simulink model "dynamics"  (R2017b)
settings: Solver=VariableStepAuto  StartTime=0.0  StopTime=10.0  RelTol=1e-3
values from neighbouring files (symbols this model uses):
  ModelInit_AngEuler = [0, 0, 0]    [Init_control.m]    (also in Init.m)
  ModelInit_PosE = [0, 0, -100]    [Init_control.m]    (also in Init.m = [0, 0, 0])
  ModelInit_Rads = 0    [Init.m]    (also in Init_control.m = 557.142)
  ModelInit_RateB = [0, 0, 0]    [Init_control.m]    (also in Init.m)
  ModelInit_VelB = [0, 0, 0]    [Init_control.m]    (also in Init.m)
  ModelParam_envGravityAcc = 9.8    [Init.m]
  ModelParam_motorCr = 1148    [Init.m]    (also in Init_control.m)
  ModelParam_motorJm = 0.0001287    [Init.m]    (also in Init_control.m)
  ModelParam_motorT = 0.02    [Init.m]    (also in Init_control.m)
  ModelParam_motorWb = -141.4    [Init.m]    (also in Init_control.m)
  ModelParam_rotorCm = 1.779e-07    [Init.m]    (also in Init_control.m)
  ModelParam_rotorCt = 1.105e-05    [Init.m]    (also in Init_control.m)
  ModelParam_uavCCm = [0.01 0.01 0.0055]    [Init.m]
  ModelParam_uavCd = 0.073    [Init.m]
  ModelParam_uavJ = [ModelParam_uavJxx, 0, 0;     0, ModelParam_uavJyy, 0;     0, 0, ModelParam_uavJzz]    [Init.m]    (also in Init_control.m)
  ModelParam_uavMass = 1.4    [Init.m]    (also in Init_control.m)
  ModelParam_uavR = 0.225    [Init.m]    (also in Init_control.m)
undefined symbols (not defined in the file or in its folder): Column, D, vector
libraries: sharedutil x2

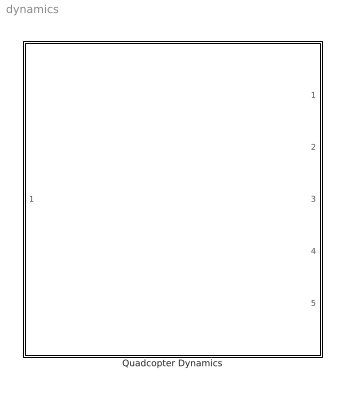
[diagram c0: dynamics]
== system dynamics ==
  Quadcopter Dynamics : Subsystem

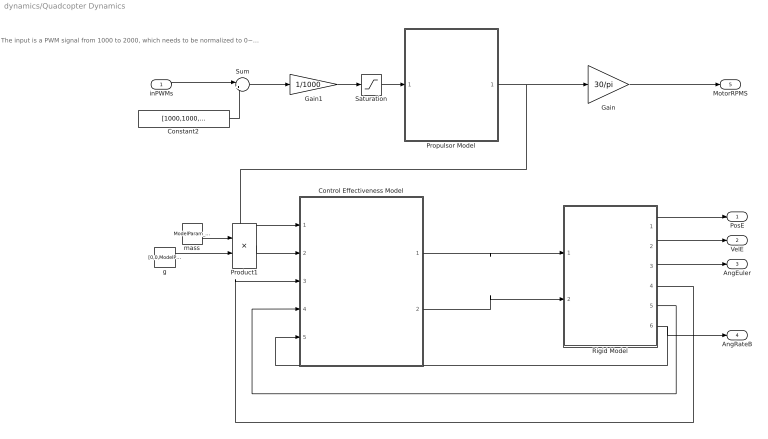
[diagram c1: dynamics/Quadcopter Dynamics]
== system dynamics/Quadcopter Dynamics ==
  note: The input is a PWM signal from 1000 to 2000, which needs to be normalized to 0~1.
  inPWMs : Inport
  Constant2 : Constant  Value=[1000,1000,1000,1000]
  Control Effectiveness Model : Subsystem
  Gain : Gain  Gain=30/pi
  Gain1 : Gain  Gain=1/1000
  Product1 : Product
  Propulsor Model : Subsystem
  Rigid Model : Subsystem
  Saturation : Saturate  UpperLimit=1  LowerLimit=0
  Sum : Sum  Inputs=|+-
  g : Constant  Value=[0,0,ModelParam_envGravityAcc]
  mass : Constant  Value=ModelParam_uavMass
  PosE : Outport
  VelE : Outport  Port=2
  AngEuler : Outport  Port=3
  AngRateB : Outport  Port=4
  MotorRPMS : Outport  Port=5
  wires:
  Saturation/1 -> Propulsor Model/1(inPWMs)
  Rigid Model/6("p,q,r ") -> Control Effectiveness Model/5(p.q,r), AngRateB/1
  mass/1 -> Product1/1
  Rigid Model/4(DCM) -> Control Effectiveness Model/3(DCM)
  Propulsor Model/1(MotorRads) -> Gain/1, Control Effectiveness Model/1(MotorRads)
  Gain1/1 -> Saturation/1
  Rigid Model/2(ve) -> VelE/1
  Sum/1 -> Gain1/1
  Product1/1 -> Control Effectiveness Model/2(mg)
  Rigid Model/5("vb ") -> Control Effectiveness Model/4(Vb)
  Rigid Model/1("xe ") -> PosE/1
  Rigid Model/3(Euler) -> AngEuler/1
  Control Effectiveness Model/1(Mb) -> Rigid Model/1(Mb)
  inPWMs/1 -> Sum/1
  Control Effectiveness Model/2(Fb) -> Rigid Model/2(f)
  Constant2/1 -> Sum/2
  g/1 -> Product1/2
  Gain/1 -> MotorRPMS/1

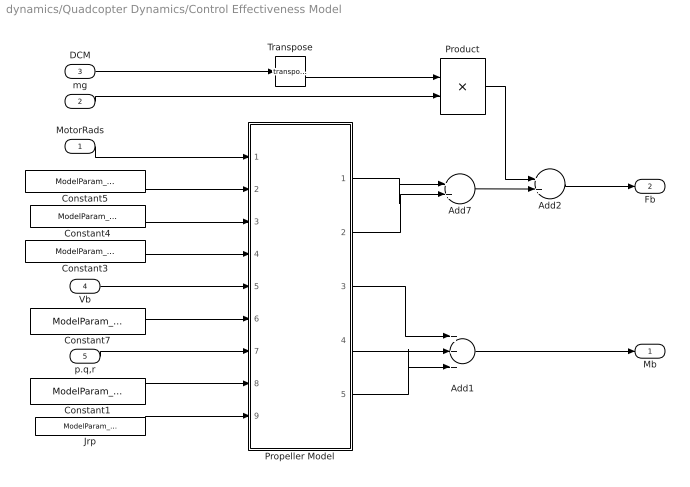
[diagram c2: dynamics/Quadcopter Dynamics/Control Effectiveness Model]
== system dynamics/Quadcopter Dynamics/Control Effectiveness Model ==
  MotorRads : Inport
  mg : Inport  Port=2
  DCM : Inport  Port=3
  Vb : Inport  Port=4
  p.q,r : Inport  Port=5
  Add1 : Sum  Inputs=+++
  Add2 : Sum
  Add7 : Sum
  Constant1 : Constant  Value=ModelParam_uavCCm
  Constant3 : Constant  Value=ModelParam_rotorCt
  Constant4 : Constant  Value=ModelParam_rotorCm
  Constant5 : Constant  Value=ModelParam_uavR
  Constant7 : Constant  Value=ModelParam_uavCd
  Jrp : Constant  Value=ModelParam_motorJm
  Product : Product  Multiplication=Matrix(*)
  Propeller Model : MATLAB Function  TreatAsAtomicUnit=on
  Transpose : Math  Operator=transpose
  Mb : Outport
  Fb : Outport  Port=2
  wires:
  Add2/1 -> Fb/1
  Constant3/1 -> Propeller Model/4(Ct)
  Propeller Model/2(Fd) -> Add7/2
  Add7/1 -> Add2/2
  Propeller Model/1(Fb) -> Add7/1
  Product/1 -> Add2/1
  mg/1 -> Product/2
  DCM/1 -> Transpose/1
  Constant7/1 -> Propeller Model/6(Cd)
  Vb/1 -> Propeller Model/5(Vb)
  Constant5/1 -> Propeller Model/2(R)
  Constant4/1 -> Propeller Model/3(Cm)
  MotorRads/1 -> Propeller Model/1(w)
  Transpose/1 -> Product/1
  Propeller Model/3(Mb) -> Add1/1
  Propeller Model/4(Md) -> Add1/2
  Add1/1 -> Mb/1
  p.q,r/1 -> Propeller Model/7(wb)
  Constant1/1 -> Propeller Model/8(Cdm)
  Jrp/1 -> Propeller Model/9(Jrp)
  Propeller Model/5(Ga) -> Add1/3

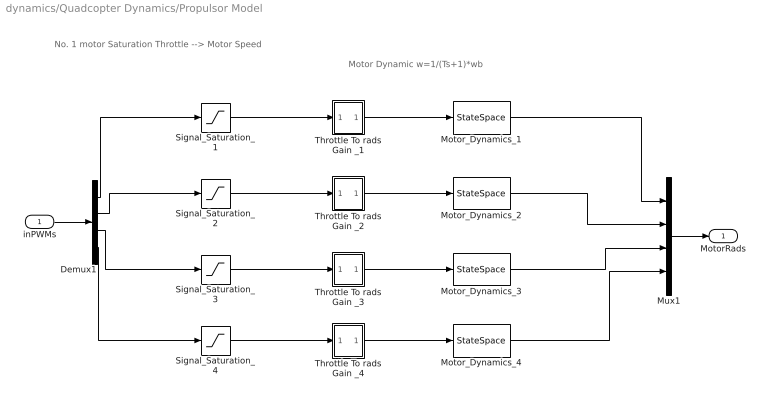
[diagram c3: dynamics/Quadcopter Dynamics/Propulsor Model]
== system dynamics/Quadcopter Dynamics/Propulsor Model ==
  note: Motor Dynamic w=1/(Ts+1)*wb
  note: No. 1 motor Saturation Throttle --> Motor Speed
  inPWMs : Inport
  Demux1 : Demux
  Motor_Dynamics_{1..4} (4 alike) : StateSpace  A=-1/ModelParam_motorT  C=1/ModelParam_motorT  D=0  InitialCondition=ModelInit_Rads*ModelParam_motorT
  Mux1 : Mux
  Signal_Saturation_{1..4} (4 alike) : Saturate  UpperLimit=1  LowerLimit=0
  Throttle To rads Gain _1 : Subsystem
  Throttle To rads Gain _2 : Subsystem
  Throttle To rads Gain _3 : Subsystem
  Throttle To rads Gain _4 : Subsystem
  MotorRads : Outport
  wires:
  Throttle To rads Gain _4/1(Out5) -> Motor_Dynamics_4/1
  Signal_Saturation_4/1 -> Throttle To rads Gain _4/1(In5)
  Signal_Saturation_3/1 -> Throttle To rads Gain _3/1(In5)
  Signal_Saturation_2/1 -> Throttle To rads Gain _2/1(In5)
  Motor_Dynamics_4/1 -> Mux1/4
  Motor_Dynamics_3/1 -> Mux1/3
  Motor_Dynamics_2/1 -> Mux1/2
  Motor_Dynamics_1/1 -> Mux1/1
  Signal_Saturation_1/1 -> Throttle To rads Gain _1/1(In5)
  Mux1/1 -> MotorRads/1
  Throttle To rads Gain _3/1(Out5) -> Motor_Dynamics_3/1
  Throttle To rads Gain _2/1(Out5) -> Motor_Dynamics_2/1
  Throttle To rads Gain _1/1(Out5) -> Motor_Dynamics_1/1
  inPWMs/1 -> Demux1/1
  Demux1/4 -> Signal_Saturation_4/1
  Demux1/3 -> Signal_Saturation_3/1
  Demux1/2 -> Signal_Saturation_2/1
  Demux1/1 -> Signal_Saturation_1/1

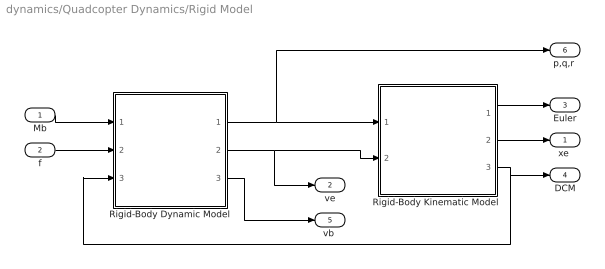
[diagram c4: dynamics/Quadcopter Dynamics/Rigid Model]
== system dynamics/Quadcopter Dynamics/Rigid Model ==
  Mb : Inport
  f : Inport  Port=2
  Rigid-Body Dynamic Model : Subsystem
  "Rigid-Body Kinematic Model " : Subsystem
  "xe " : Outport
  ve : Outport  Port=2
  Euler : Outport  Port=3
  DCM : Outport  Port=4
  "vb " : Outport  Port=5
  "p,q,r " : Outport  Port=6
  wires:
  Rigid-Body Dynamic Model/1("p,q,r ") -> "Rigid-Body Kinematic Model "/1(pqr), "p,q,r "/1
  "Rigid-Body Kinematic Model "/1(Euler) -> Euler/1
  "Rigid-Body Kinematic Model "/3(DCM) -> Rigid-Body Dynamic Model/3(DCM), DCM/1
  Mb/1 -> Rigid-Body Dynamic Model/1(Mb)
  f/1 -> Rigid-Body Dynamic Model/2(f)
  Rigid-Body Dynamic Model/2(ve) -> "Rigid-Body Kinematic Model "/2(ve), ve/1
  Rigid-Body Dynamic Model/3("vb ") -> "vb "/1
  "Rigid-Body Kinematic Model "/2("xe ") -> "xe "/1

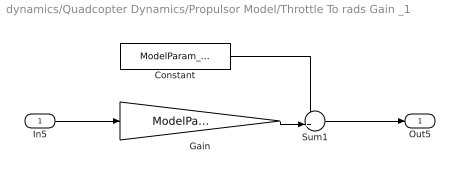
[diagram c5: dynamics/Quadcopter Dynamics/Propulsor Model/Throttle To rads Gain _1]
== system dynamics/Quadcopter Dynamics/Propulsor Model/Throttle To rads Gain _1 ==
  In5 : Inport
  Constant : Constant  Value=ModelParam_motorWb
  Gain : Gain  Gain=ModelParam_motorCr
  Sum1 : Sum  Inputs=++|
  Out5 : Outport
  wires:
  Constant/1 -> Sum1/1
  Gain/1 -> Sum1/2
  In5/1 -> Gain/1
  Sum1/1 -> Out5/1

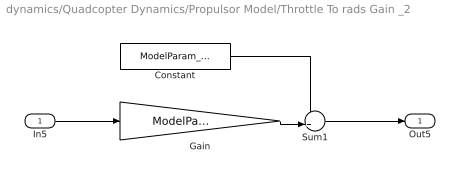
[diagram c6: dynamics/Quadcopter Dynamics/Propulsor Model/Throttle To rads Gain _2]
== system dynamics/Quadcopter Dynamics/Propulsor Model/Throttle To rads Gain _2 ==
  In5 : Inport
  Constant : Constant  Value=ModelParam_motorWb
  Gain : Gain  Gain=ModelParam_motorCr
  Sum1 : Sum  Inputs=++|
  Out5 : Outport
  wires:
  Sum1/1 -> Out5/1
  In5/1 -> Gain/1
  Gain/1 -> Sum1/2
  Constant/1 -> Sum1/1

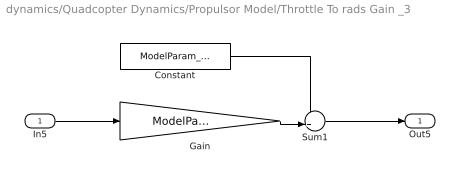
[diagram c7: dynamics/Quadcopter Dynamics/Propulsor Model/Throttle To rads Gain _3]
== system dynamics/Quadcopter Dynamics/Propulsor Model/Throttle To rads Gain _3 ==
  In5 : Inport
  Constant : Constant  Value=ModelParam_motorWb
  Gain : Gain  Gain=ModelParam_motorCr
  Sum1 : Sum  Inputs=++|
  Out5 : Outport
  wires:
  Constant/1 -> Sum1/1
  Gain/1 -> Sum1/2
  In5/1 -> Gain/1
  Sum1/1 -> Out5/1

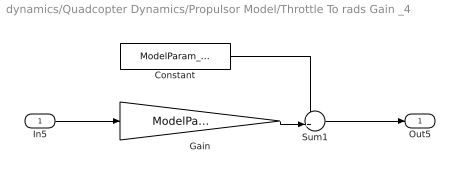
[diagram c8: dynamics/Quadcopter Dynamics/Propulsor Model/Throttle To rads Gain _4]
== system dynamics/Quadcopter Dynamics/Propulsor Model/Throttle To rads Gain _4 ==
  In5 : Inport
  Constant : Constant  Value=ModelParam_motorWb
  Gain : Gain  Gain=ModelParam_motorCr
  Sum1 : Sum  Inputs=++|
  Out5 : Outport
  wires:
  Sum1/1 -> Out5/1
  In5/1 -> Gain/1
  Gain/1 -> Sum1/2
  Constant/1 -> Sum1/1

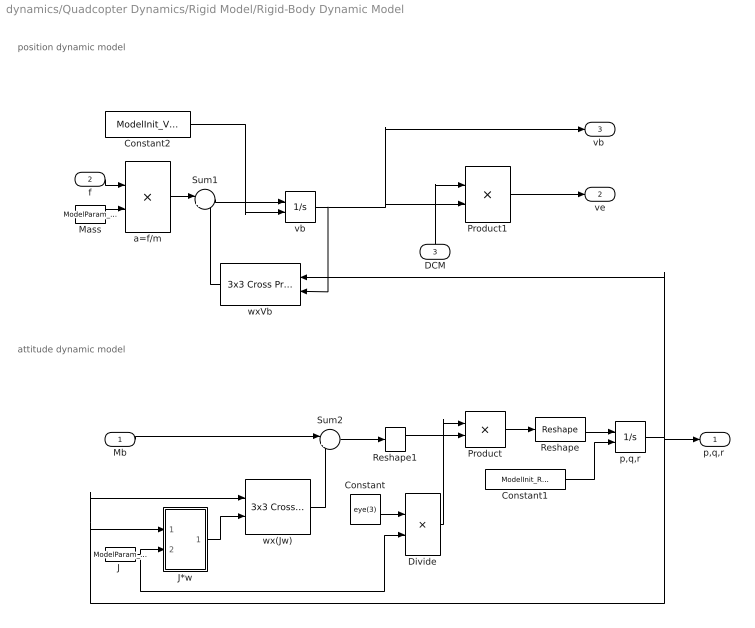
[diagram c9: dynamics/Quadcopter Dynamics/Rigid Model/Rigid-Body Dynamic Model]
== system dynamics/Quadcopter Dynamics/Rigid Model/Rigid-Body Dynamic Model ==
  note: attitude dynamic model
  note: position dynamic model
  Mb : Inport
  f : Inport  Port=2
  DCM : Inport  Port=3
  " Mass " : Constant  Value=ModelParam_uavMass
  Constant : Constant  Value=eye(3)
  Constant1 : Constant  Value=ModelInit_RateB
  Constant2 : Constant  Value=ModelInit_VelB
  Divide : Product  Inputs=*/  Multiplication=Matrix(*)
  "J " : Constant  Value=ModelParam_uavJ
  J*w : Subsystem
  Product : Product  Multiplication=Matrix(*)
  Product1 : Product  Multiplication=Matrix(*)
  Reshape : Reshape  OutputDimensionality=Customize  OutputDimensions=[3,1]
  Reshape1 : Reshape  OutputDimensionality=Column vector (2-D)
  Sum1 : Sum  Inputs=|+-
  Sum2 : Sum  Inputs=|+-
  a=f/m : Product  Inputs=*/
  p,q,r : Integrator  InitialConditionSource=external
  vb : Integrator  InitialConditionSource=external
  wx(Jw) : sharedutil/3x3 Cross Product
  wxVb : sharedutil/3x3 Cross Product
  "p,q,r " : Outport
  ve : Outport  Port=2
  "vb " : Outport  Port=3
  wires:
  Product/1 -> Reshape/1
  Reshape1/1 -> Product/2
  Constant/1 -> Divide/1
  Divide/1 -> Product/1
  Sum2/1 -> Reshape1/1
  "J "/1 -> Divide/2, J*w/2(J)
  p,q,r/1 -> "p,q,r "/1, J*w/1(p q r), wx(Jw)/1, wxVb/1
  J*w/1("J*w ") -> wx(Jw)/2
  Mb/1 -> Sum2/1
  wx(Jw)/1 -> Sum2/2
  Constant2/1 -> vb/2
  f/1 -> a=f/m/1
  Product1/1 -> ve/1
  wxVb/1 -> Sum1/2
  a=f/m/1 -> Sum1/1
  Sum1/1 -> vb/1
  vb/1 -> Product1/2, "vb "/1, wxVb/2
  " Mass "/1 -> a=f/m/2
  DCM/1 -> Product1/1
  Reshape/1 -> p,q,r/1
  Constant1/1 -> p,q,r/2

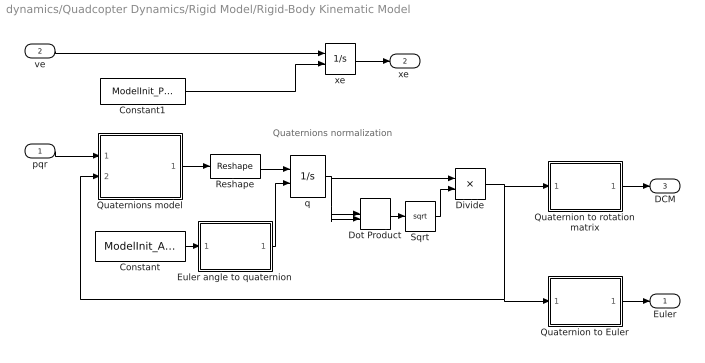
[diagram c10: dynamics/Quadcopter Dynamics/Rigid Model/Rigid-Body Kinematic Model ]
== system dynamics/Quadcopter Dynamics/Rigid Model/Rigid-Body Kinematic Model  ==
  note: Quaternions normalization
  pqr : Inport
  ve : Inport  Port=2
  Constant : Constant  Value=ModelInit_AngEuler
  Constant1 : Constant  Value=ModelInit_PosE
  Divide : Product  Inputs=*/
  Dot Product : DotProduct
  Euler angle to quaternion : MATLAB Function
  Quaternion to Euler : MATLAB Function
  Quaternion to rotation matrix : MATLAB Function
  Quaternions model : MATLAB Function  TreatAsAtomicUnit=on
  Reshape : Reshape  OutputDimensionality=Customize  OutputDimensions=[4,1]
  Sqrt : Sqrt
  q : Integrator  InitialConditionSource=external
  xe : Integrator  InitialConditionSource=external
  Euler : Outport
  "xe " : Outport  Port=2
  DCM : Outport  Port=3
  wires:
  Divide/1 -> Quaternion to rotation matrix/1(q), Quaternions model/2(q), Quaternion to Euler/1(q)
  Dot Product/1 -> Sqrt/1
  pqr/1 -> Quaternions model/1(pqr)
  q/1 -> Divide/1, Dot Product/1, Dot Product/2
  Quaternions model/1(qdot) -> Reshape/1
  Quaternion to rotation matrix/1(Reb) -> DCM/1
  Quaternion to Euler/1(y) -> Euler/1
  Constant/1 -> Euler angle to quaternion/1(EulerAngle)
  Euler angle to quaternion/1(q) -> q/2
  Reshape/1 -> q/1
  ve/1 -> xe/1
  xe/1 -> "xe "/1
  Constant1/1 -> xe/2
  Sqrt/1 -> Divide/2

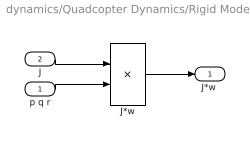
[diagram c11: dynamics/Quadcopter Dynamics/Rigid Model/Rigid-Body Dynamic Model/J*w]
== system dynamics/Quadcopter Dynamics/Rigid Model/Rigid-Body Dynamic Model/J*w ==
  p q r : Inport
  J : Inport  Port=2
  J*w : Product  Multiplication=Matrix(*)
  "J*w " : Outport
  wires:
  J*w/1 -> "J*w "/1
  J/1 -> J*w/1
  p q r/1 -> J*w/2

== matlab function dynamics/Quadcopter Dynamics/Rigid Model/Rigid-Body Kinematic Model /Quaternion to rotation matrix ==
function Reb = fcn(q)
%Function description;
%  The rotation matrix of the Aircraft-Body Coordinate Frame (ABCF) to the
%  Earth-Fixed Coordinate Frame (EFCF) is obtained from the quaternions
Reb = [q(1)*q(1) + q(2)*q(2) - q(3)*q(3) - q(4)*q(4), 2*(q(2)*q(3) - q(1)*q(4)), 2*(q(2)*q(4) + q(1)*q(3))
           2*(q(2)*q(3) + q(1)*q(4)), q(1)*q(1) - q(2)*q(2) + q(3)*q(3) - q(4)*q(4), 2*(q(3)*q(4) - q(1)*q(2))
           2*(q(2)*q(4) - q(1)*q(3)), 2*(q(3)*q(4) + q(1)*q(2)), q(1)*q(1) - q(2)*q(2) - q(3)*q(3) + q(4)*q(4)];

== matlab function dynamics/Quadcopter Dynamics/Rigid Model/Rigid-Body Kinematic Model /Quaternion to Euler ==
function y = fcn(q)
 %Function description:
%  Quaternions to Euler
phi = atan2(2*(q(1)*q(2) + q(3)*q(4)), (1 - 2*(q(2)*q(2) + q(3)*q(3))));
theta = asin(2*(q(1)*q(3) - q(2)*q(4)));
psi = atan2(2*(q(1)*q(4) + q(2)*q(3)), (1 - 2*(q(3)*q(3) + q(4)*q(4))));
y = [phi theta psi];

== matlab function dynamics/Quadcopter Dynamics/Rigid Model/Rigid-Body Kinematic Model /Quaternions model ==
function qdot = fcn(pqr, q)
%Function description:
%  Quaternions model
qdot = 0.5*[0, -pqr(1), -pqr(2), -pqr(3); pqr(1), 0, pqr(3), -pqr(2); pqr(2), -pqr(3), 0, pqr(1); pqr(3), pqr(2), -pqr(1), 0]*q;

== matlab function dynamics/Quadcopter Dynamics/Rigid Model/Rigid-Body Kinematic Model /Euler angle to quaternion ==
function q = fcn(EulerAngle)
%Function description:
%  Get quaternions from Euler angle
q0 =  cos(EulerAngle(1)/2)*cos(EulerAngle(2)/2)*cos(EulerAngle(3)/2) + sin(EulerAngle(1)/2)*sin((EulerAngle(2)/2))*sin((EulerAngle(3)/2));
q1 = sin(EulerAngle(1)/2)*cos(EulerAngle(2)/2)*cos(EulerAngle(3)/2) - cos(EulerAngle(1)/2)*sin((EulerAngle(2)/2))*sin((EulerAngle(3)/2));
q2 = cos(EulerAngle(1)/2)*sin(EulerAngle(2)/2)*cos(EulerAngle(3)/2) + sin(EulerAngle(1)/2)*cos((EulerAngle(2)/2))*sin((EulerAngle(3)/2));
q3 = cos(EulerAngle(1)/2)*cos(EulerAngle(2)/2)*sin(EulerAngle(3)/2) - sin(EulerAngle(1)/2)*sin((EulerAngle(2)/2))*cos((EulerAngle(3)/2));
q = [q0 q1 q2 q3]';

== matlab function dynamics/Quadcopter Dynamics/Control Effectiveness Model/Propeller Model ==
function [Fb, Fd, Mb, Md, Ga] = fcn(w, R, Cm, Ct, Vb, Cd,wb, Cdm, Jrp)
 %Function description:
 %  Obtain the force and torque acting on the body. The airframe of the
 %  quadrotor is as follows:
 %3↓   1↑
 %  \ /
 %  / \
 %2↑   4↓
 %↑ stands for counterclockwise and ↓stands for clockwise.
 %Input：
 %  w: motor speed，unit：rad/s
 %  R: body radius(m)
 %  Cm: torque coefficient
 %  Ct: thrust coefficient
 %  Vb: aircraft speed in the body coordinate system
 %  Cd: damping coefficient
 %  wb: angular velocity in the body coordinate system
 %  Cdm: damping moment coefficient vector
 %  Jrp:  moment of inertia of motor rotor + propeller
 %Output:
 %  Fb: thrust under the body coordinate system
 %  Fd: aerodynamic force under the body coordinate system
 %  Mb: torque under the body coordinate system
 %  Md: aerodynamic moment
 %  Ga: gyro moment
 M_rctcm = [-sin(pi/4)*R*Ct, sin(pi/4)*R*Ct, sin(pi/4)*R*Ct, -sin(pi/4)*R*Ct;
            sin(pi/4)*R*Ct, -sin(pi/4)*R*Ct, sin(pi/4)*R*Ct, -sin(pi/4)*R*Ct;
            Cm, Cm, -Cm, -Cm];
 Mb = M_rctcm*(w.^2);  % torque
 
 Fb = [0; 0; -sum(Ct*(w.^2))];  % thrust
 Fd = -Cd*Vb.*abs(Vb)*0.5;  % aerodynamic force
 Md = -Cdm.*wb.*abs(wb);  % aerodynamic moment
 % gyro moment
 Ga = zeros(3,1);
 Ga(1) = Jrp*wb(2)*( w(1) + w(2) - w(3) - w(4));
 Ga(2) = Jrp*wb(1)*(-w(1) - w(2) + w(3) + w(4));
end
